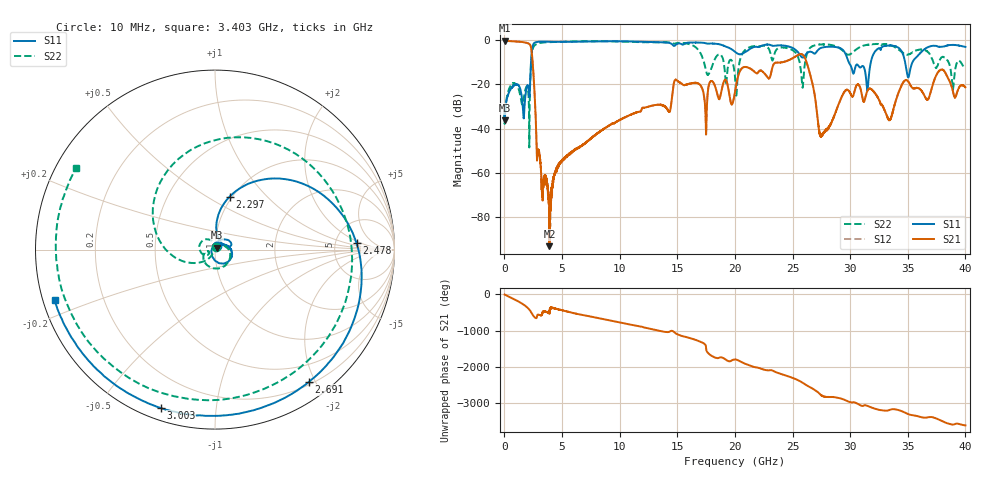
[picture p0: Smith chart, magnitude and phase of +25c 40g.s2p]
!Keysight Technologies,N5234A,MY52241180,A.10.60.03
!Date: Thursday, February 22, 2024 16:23:14
!Correction: S11(Full 2 Port(1,2))
!S21(Full 2 Port(1,2))
!S12(Full 2 Port(1,2))
!S22(Full 2 Port(1,2))
!S2P File: Measurements: S11, S21, S12, S22:
# Hz S  dB  R 50
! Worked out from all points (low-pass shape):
!   6401 points, 10 MHz to 40 GHz, reference 50 ohm
!   highest |S21| = -0.07 dB at 10 MHz (marker M1); lowest = -93.3 dB at 3.903 GHz (marker M2)
!   |S21| within 3 dB of the highest: start of sweep to 2.295 GHz
!   lowest |S11| = -36.2 dB at 16.25 MHz (marker M3), VSWR 1.03, Z = 51.2 + j1.06 ohm
!   |S11| at or under -10 dB: start of sweep to 2.3 GHz; 29.89 GHz to 31.79 GHz (1.9 GHz wide, 6.16 % of centre); 34.77 GHz to 35.4 GHz (627.5 MHz wide, 1.79 % of centre)
!   |S22| runs from -48.5 to -0.4 dB; largest |S21 - S12| = 0.0098
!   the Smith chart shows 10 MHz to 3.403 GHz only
!   S11 on the Smith chart (normalised r, x): 10 MHz: 1.02, +0.04; 2.297 GHz: 0.97, +0.63; 2.478 GHz: 8.21, +1.54; 2.691 GHz: 0.24, -1.92; 3.003 GHz: 0.05, -0.71; 3.403 GHz: 0.03, -0.15
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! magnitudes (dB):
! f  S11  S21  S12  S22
! 10 MHz  -32.3  -0.1  0.0  -35.1
! 16.25 MHz  -36.2  -0.1  -0.1  -37.9
! 666.1 MHz  -21.3  -0.4  -0.4  -19.8
! 1.691 GHz  -34.6  -0.9  -0.9  -25.6
! 2.297 GHz  -10.3  -3.1  -3.1  -11.2
! 2.478 GHz  -2.1  -12.4  -12.4  -3.4
! 2.691 GHz  -0.9  -32.7  -32.8  -2.0
! 3.003 GHz  -0.6  -50.5  -50.1  -1.2
! 3.403 GHz  -0.6  -65.3  -63.5  -0.9
! 3.903 GHz  -0.6  -93.3  -82.6  -0.8
! 6.677 GHz  -0.6  -47.8  -47.8  -0.5
! 13.34 GHz  -0.8  -29.2  -29.2  -0.9
! 14.92 GHz  -1.8  -18.0  -18.0  -1.3
! 20 GHz  -5.2  -23.4  -23.4  -16.6
! 21.6 GHz  -3.1  -13.8  -13.8  -2.6
! 25.65 GHz  -6.7  -6.3  -6.2  -11.1
! 26.67 GHz  -5.3  -18.4  -18.4  -2.8
! 27.51 GHz  -3.4  -43.3  -43.6  -1.8
! 30.65 GHz  -11.1  -20.0  -20.0  -3.7
! 33.34 GHz  -2.3  -35.7  -35.7  -2.0
! 34.79 GHz  -10.5  -18.1  -18.1  -6.3
! 40 GHz  -3.0  -21.3  -21.3  -11.5
